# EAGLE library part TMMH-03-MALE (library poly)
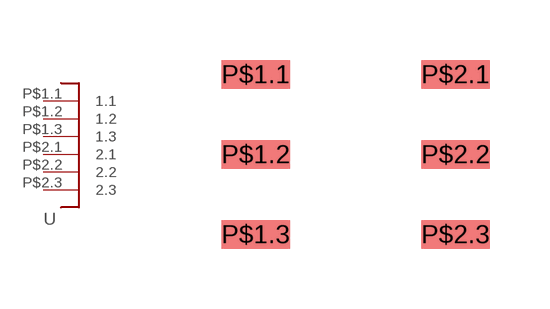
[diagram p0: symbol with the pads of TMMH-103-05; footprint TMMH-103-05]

Designator prefix -

## TMMH-03-MALE  [TMMH-103-05]
P$1.1  1.1
P$1.2  1.2
P$1.3  1.3
P$2.1  2.1
P$2.2  2.2
P$2.3  2.3

## Footprint TMMH-103-05 (pad centres in mm)
smd 1.724 x 0.72: P$1.1 -2.5,2; P$1.2 -2.5,0; P$1.3 -2.5,-2; P$2.1 2.5,2; P$2.2 2.5,0; P$2.3 2.5,-2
